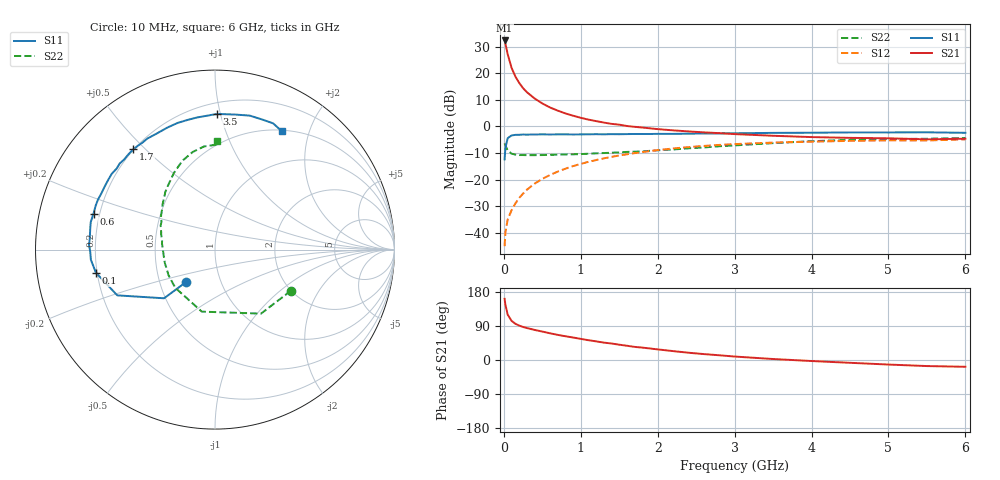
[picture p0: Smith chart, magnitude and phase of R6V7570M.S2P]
! SIEMENS Small Signal Semiconductors
! BFR193
! Si NPN RF Bipolar Junction Transistor in SOT23
! VCE = 0.75 V  IC = 70 mA
! Common Emitter S-Parameters:  May  1996
# GHz  S  MA  R  50
!  f  S11  S21  S12  S22
! GHz  MAG  ANG  MAG  ANG  MAG  ANG  MAG  ANG
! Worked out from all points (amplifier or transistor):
!   36 points, 10 MHz to 6 GHz, reference 50 ohm
!   highest |S21| = 32.3 dB at 10 MHz (marker M1)
!   |S21| within 3 dB of that: start of sweep to 33.84 MHz
!   unconditionally stable (mu >= 1): start of sweep to 19.51 MHz; 116 MHz to end of sweep
!   at 250 MHz: K = 1.12, MAG = 17.7 dB, |S12| = -25.3 dB
!   at 1.4 GHz: K = 1.10, MAG = 4.3 dB, |S12| = -11.5 dB
!   at 6 GHz: K = 1.03, MAG = -0.9 dB, |S12| = -4.9 dB
!   S11 on the Smith chart (normalised r, x): 10 MHz: 0.68, -0.26; 100 MHz: 0.20, -0.09; 600 MHz: 0.18, +0.14; 1.7 GHz: 0.20, +0.46; 3.5 GHz: 0.28, +0.98; 6 GHz: 0.51, +1.59
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0.01  0.24 -131.6  41.33 161.5  0.0056 62.1  0.4809 -28.5
0.02  0.3926 -136.3  36.31 146.0  0.0101 62.6  0.4392 -54.3
0.05  0.6011 -154.9  22.73 119.7  0.0178 58.0  0.3534 -102.0
0.1  0.6758 -169.0  12.67 103.3  0.0265 62.2  0.307 -136.2
0.15  0.6939 -175.3  8.676 95.6  0.0356 65.9  0.2957 -151.1
0.2  0.6955 -179.3  6.572 90.8  0.0453 68.5  0.2894 -159.0
0.25  0.7028 177.8  5.239 87.1  0.0545 70.4  0.2894 -164.8
0.3  0.7003 175.4  4.395 84.4  0.0646 71.1  0.288 -168.5
0.4  0.7048 170.5  3.352 79.4  0.084 71.3  0.288 -174.0
0.5  0.7091 167.5  2.703 75.0  0.103 70.9  0.2893 -178.3
0.6  0.7058 163.5  2.27 70.5  0.1221 69.6  0.2912 178.4
0.7  0.7086 159.7  1.982 66.3  0.1413 68.4  0.2944 175.8
0.8  0.7089 156.8  1.755 62.7  0.1601 66.6  0.2975 173.3
1.1  0.7105 147.0  1.343 52.2  0.2158 61.3  0.3068 166.4
1.3  0.71 140.5  1.181 45.9  0.2509 57.5  0.3156 161.8
1.7  0.7206 129.1  0.983 34.6  0.3144 49.8  0.3347 153.4
2.2  0.7237 116.4  0.843 23.5  0.3845 40.0  0.3679 143.5
3  0.7427 97.9  0.717 9.1  0.4654 25.0  0.4391 127.1
3.5  0.7559 89.2  0.667 2.6  0.4962 16.7  0.4852 118.1
4.5  0.7712 75.5  0.609 -7.4  0.5345 3.2  0.5581 102.8
5.5  0.7744 65.3  0.571 -16.0  0.5447 -8.7  0.5863 88.3
6  0.758 60.7  0.588 -17.9  0.5702 -12.4  0.6052 88.9
